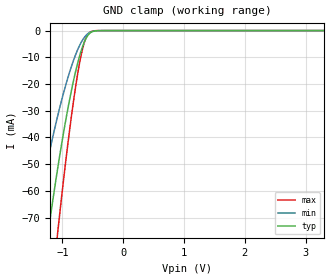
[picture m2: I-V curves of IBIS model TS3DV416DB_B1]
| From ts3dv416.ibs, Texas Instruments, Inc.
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[Model]   TS3DV416DB_B1
Model_type  Terminator
| variable   typ   min   max
C_comp   2.60pF   2.20pF   2.89pF
| C_tri-state   2.60pF   2.20pF   2.89pF
[Temperature Range]   40   100   -40
| Ambient temperature   25   85   -40
[Voltage range]   3.3   3   3.6
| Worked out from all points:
|   GND clamp passes 1 mA (typ) near -0.55 V on its own axis
[GND Clamp]
| TS3DV416DB_B1
|   Voltage   I(typ)   I(min)   I(max)
-3.3V     -516.6mA   -373.8mA   -672.1mA
-1.485V   -119.1mA   -77.22mA   -171mA
-1.445V   -111.8mA   -72.2mA    -161mA
-1.24V    -76.46mA   -48.32mA   -111.6mA
-1.205V   -70.84mA   -44.58mA   -103.6mA
-1.08V    -51.84mA   -32.12mA   -76.04mA
-885mV    -26.22mA   -15.78mA   -37.81mA
-745mV    -11.82mA   -6.937mA   -15.61mA
-685mV    -7.072mA   -4.161mA   -8.448mA
-635mV    -4.005mA   -2.424mA   -4.145mA
-525mV    -594.7uA   -446uA     -344.6uA
3.3V      199.2pA    823.5pA    19.61pA
